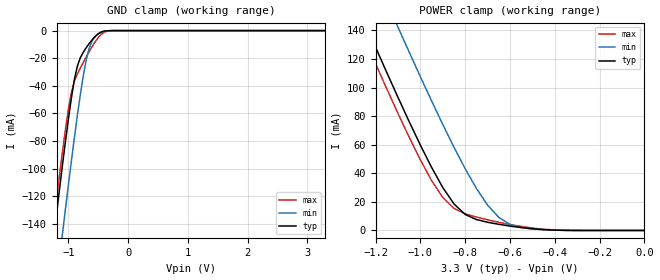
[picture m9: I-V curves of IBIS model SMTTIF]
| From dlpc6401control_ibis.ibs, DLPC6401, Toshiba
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[Model]   SMTTIF
Model_type   Input
Polarity   Non-Inverting
Vinl =   0.8000V
Vinh =   2.0000V
C_comp   1.443pF   NA   NA
|Variable   typ   min   max
[Voltage range]  3.3   3.0   3.6
[Temperature Range]   25.0000   125.000   0.000
[POWER Clamp Reference]   3.3000V   3.0000V   3.6000V
[GND Clamp Reference]   0.000V   0.000V   0.000V
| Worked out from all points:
|   GND clamp passes 1 mA (typ) near -0.45 V on its own axis
|   POWER clamp passes 1 mA (typ) near -0.48 V on its own axis
[GND_clamp]
| voltage   I(typ)   I(min)   I(max)
-3.3V     -944.9mA   -993.6mA   -933.7mA
-1.3V     -169.6mA   -220.5mA   -158.5mA
-1.25V    -151.2mA   -201.9mA   -140.2mA
-1.2V     -132.9mA   -183.4mA   -122.2mA
-1.1V     -97.21mA   -147mA     -87.47mA
-1V       -63.63mA   -111.4mA   -56.62mA
-900mV    -35.29mA   -77.26mA   -36.39mA
-800mV    -19.53mA   -45.93mA   -27.04mA
-700mV    -12.2mA    -20.73mA   -18.85mA
-600mV    -6.422mA   -7.153mA   -11.28mA
-450mV    -954.9uA   -1.183mA   -2.691mA
3.3V      2.122nA    24.26uA    12.22nA
[POWER_clamp]
| voltage   I(typ)   I(min)   I(max)
-3.3V     917.5mA    964.8mA    906.4mA
-1.3V     164.1mA    213.9mA    152.5mA
-1.25V    146mA      195.8mA    134.5mA
-1.2V     128.2mA    177.9mA    116.7mA
-1.1V     93.14mA    142.3mA    81.92mA
-950mV    44.15mA    90.68mA    34.95mA
-850mV    18.58mA    58.26mA    15.44mA
-750mV    7.652mA    29.46mA    9.374mA
-650mV    4.312mA    9.163mA    5.736mA
-600mV    3.088mA    4.252mA    4.184mA
-500mV    1.206mA    1.062mA    1.712mA
0V        2.122nA    56.31nA    15.39nA
